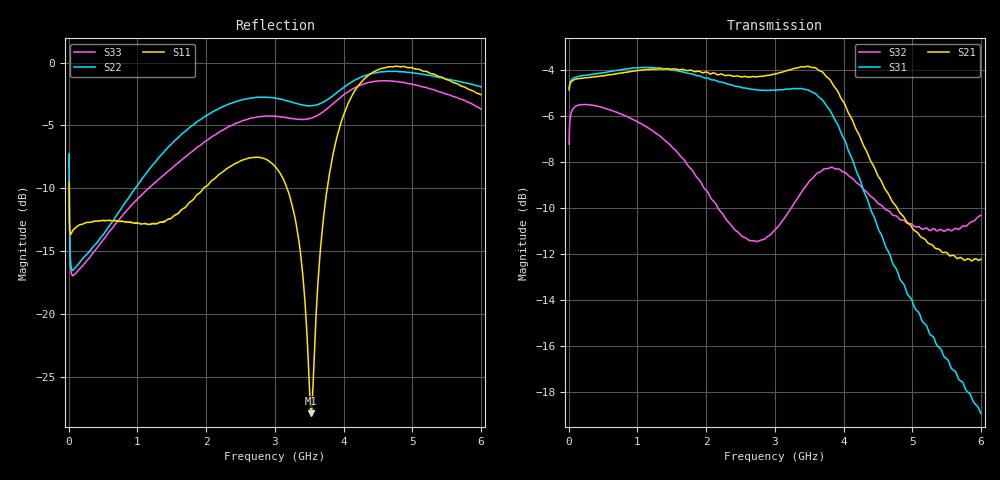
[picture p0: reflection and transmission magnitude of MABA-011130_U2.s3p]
!Agilent Technologies,E5071C,MY46110647,A.11.31
!Date: Fri Mar 25 10:16:56 2022 DD
!Data & Calibration Information:
!MABA-011130 soldered onto PT-0028476 with SMA connectors, Calibration PCB, Port1 (pin1) Port2 (pin2) Port3 (pin3)
!Freq	S11:SOLT3(ON)	S12:SOLT3(ON)	S13:SOLT3(ON)
!	S21:SOLT3(ON)	S22:SOLT3(ON)	S23:SOLT3(ON)
!	S31:SOLT3(ON)	S32:SOLT3(ON)	S33:SOLT3(ON)
!PortZ  Port1:50+j0  Port2:50+j0  Port3:50+j0
!Above PortZ is port z conversion or system Z0 setting when saving the data.
!When reading, reference impedance value at option line is always used.
# Hz S MA R 50
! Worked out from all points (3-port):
!   1200 points, 5 MHz to 6 GHz, reference 50 ohm
!   strongest paths, dB at 5 MHz, 1.505 GHz, 3.005 GHz, 4.505 GHz, 6 GHz:
!     S21: -4.9, -4.0, -4.2, -8.6, -12.2
!     S31: -4.8, -4.0, -4.9, -10.9, -18.9
!     S32: -7.2, -7.4, -10.9, -9.8, -10.3
!   lowest |S11| = -27.9 dB at 3.53 GHz (marker M1), VSWR 1.08, Z = 51.5 + j3.8 ohm
!   |S11| at or under -10 dB: 5.765 MHz to 1.962 GHz (1.957 GHz wide, 199 % of centre); 3.179 GHz to 3.763 GHz (583.4 MHz wide, 16.8 % of centre)
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5000000  0.3347 71.3  0.5661 -164.3  0.5704 15.3
         0.5705 -164.2  0.4349 103.8  0.4342 36.8
         0.5754 15.4  0.4345 36.8  0.4295 103.7
7.5e7  0.2174 4.6  0.6001 175.8  0.6057 -3.7
       0.5998 175.8  0.1509 23.9  0.5217 -0.0
       0.6057 -3.7  0.5218 -0.0  0.1429 19.7
1.22e9  0.2292 -81.8  0.6382 79.3  0.6405 -95.5
        0.6329 79.6  0.3913 -50.5  0.4693 -73.5
        0.6375 -96.4  0.465 -73.1  0.3269 -78.3
2.11e9  0.3434 -107.0  0.6165 3.5  0.5992 -171.3
        0.6211 4.5  0.6403 -96.1  0.3291 -122.3
        0.5992 -170.9  0.3266 -121.8  0.5122 -111.1
3.005e9  0.3861 -163.1  0.6197 -69.5  0.5662 112.3
         0.6176 -70.1  0.7218 -138.7  0.2902 -146.6
         0.5695 112.1  0.2836 -147.8  0.6114 -144.4
3.335e9  0.2079 164.8  0.6438 -100.2  0.5702 79.5
         0.637 -100.7  0.6857 -145.7  0.3405 -162.8
         0.5739 79.3  0.3323 -163.8  0.5949 -149.1
3.53e9  0.04026 66.0  0.6471 -120.6  0.5607 57.8
        0.6382 -121.2  0.6734 -145.6  0.3728 -176.9
        0.5651 57.5  0.3643 -177.9  0.6009 -148.1
3.845e9  0.4288 -49.4  0.5932 -154.8  0.4967 21.2
         0.5858 -155.9  0.7378 -143.1  0.3934 156.1
         0.5007 20.1  0.3863 155.2  0.6851 -146.7
4.5e9  0.9353 -104.3  0.377 150.4  0.2897 -40.0
       0.3713 150.2  0.9135 -154.4  0.3235 109.4
       0.2861 -40.2  0.3233 109.2  0.8439 -161.1
6e9  0.7451 179.1  0.2343 84.8  0.1098 -114.6
     0.2445 84.1  0.8004 161.0  0.2992 46.6
     0.113 -112.7  0.3044 46.5  0.652 141.5
